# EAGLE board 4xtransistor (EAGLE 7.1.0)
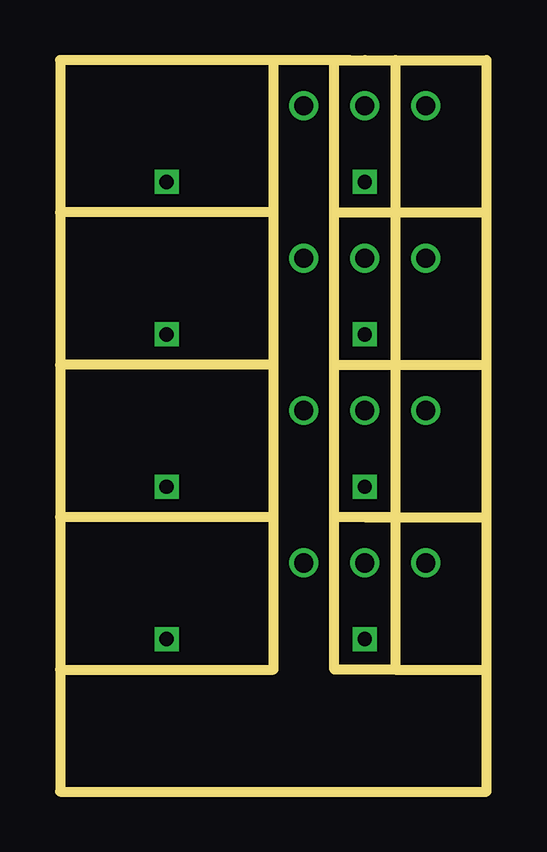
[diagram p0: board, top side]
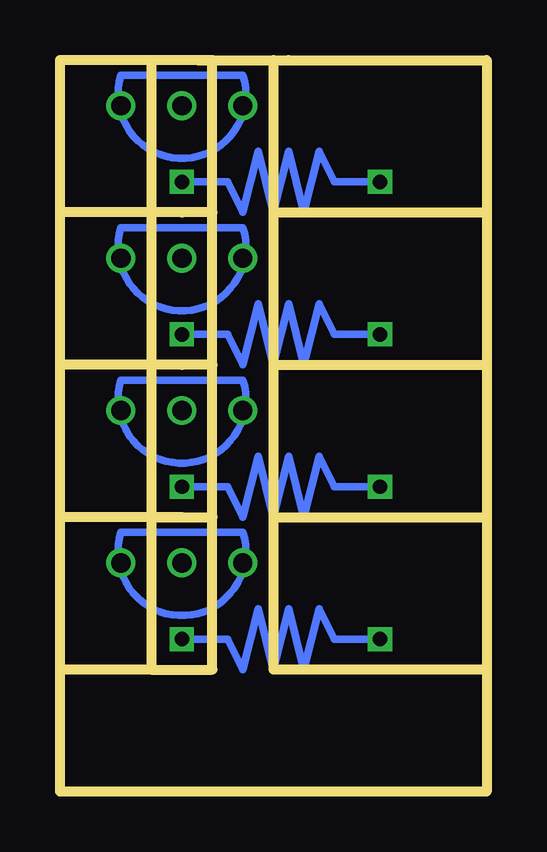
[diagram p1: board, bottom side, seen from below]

Size 17.78 x 30.48 mm. Coordinates in mm from the lower left corner, seen from the top.
Outline: 47 segments
Copper layers (1*16): Top 0.035mm / dielectric 1.5mm / Bottom 0.035mm
Design rules "default": minimum track width 10mil, minimum drill 24mil, track to track 8mil, track to pad 8mil, pad to pad 8mil, via to via 8mil, smd to smd 8mil, copper to edge 40mil, drill to drill 8mil, minimum pad ring 10mil, minimum via ring 8mil, stop-mask expansion 4mil, vias tented up to drill 0mil, thermal gap 10mil

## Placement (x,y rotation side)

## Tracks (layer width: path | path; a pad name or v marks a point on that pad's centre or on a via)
S$2  (via drill 0.8)
  other vias: 15.24,9.53
S$3
  Bottom 0.305: 10.16,10.79 15.24,10.79 arc-215 10.16,10.79
S$4  (via drill 0.8)
  other vias: 12.7,9.53
S$5
  Bottom 0.305: 10.16,17.14 15.24,17.14 arc-215 10.16,17.14
S$6  (via drill 0.8)
  other vias: 15.24,15.88
S$7
  Bottom 0.305: 10.16,23.5 15.24,23.5 arc-215 10.16,23.5
S$8  (via drill 0.8)
  other vias: 12.7,22.23
S$9
  Bottom 0.305: 10.16,29.84 15.24,29.84 arc-215 10.16,29.84
S$10  (via drill 0.8)
  other vias: 12.7,28.57
S$11  (via drill 0.8)
  other vias: 10.16,9.53
S$12  (via drill 0.8)
  other vias: 10.16,15.88
S$13  (via drill 0.8)
  other vias: 12.7,15.88
S$14  (via drill 0.8)
  other vias: 15.24,22.23
S$15  (via drill 0.8)
  other vias: 10.16,22.23
S$16  (via drill 0.8)
  other vias: 15.24,28.57
S$17  (via drill 0.6)
  Bottom 0.305: v12.7,6.35 10.79,6.35 10.16,5.08 9.53,7.62 8.89,5.08 8.26,7.62 7.62,5.08 6.99,7.62 6.35,6.35 v4.45,6.35
S$18  (via drill 0.6)
  Bottom 0.305: v12.7,12.7 10.79,12.7 10.16,11.43 9.53,13.97 8.89,11.43 8.26,13.97 7.62,11.43 6.99,13.97 6.35,12.7 v4.45,12.7
S$19  (via drill 0.8)
  other vias: 10.16,28.57
S$20  (via drill 0.6)
  Bottom 0.305: v12.7,19.05 10.79,19.05 10.16,17.78 9.53,20.32 8.89,17.78 8.26,20.32 7.62,17.78 6.99,20.32 6.35,19.05 v4.45,19.05
S$25  (via drill 0.6)
  Bottom 0.305: v12.7,25.4 10.79,25.4 10.16,24.13 9.53,26.67 8.89,24.13 8.26,26.67 7.62,24.13 6.99,26.67 6.35,25.4 v4.45,25.4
